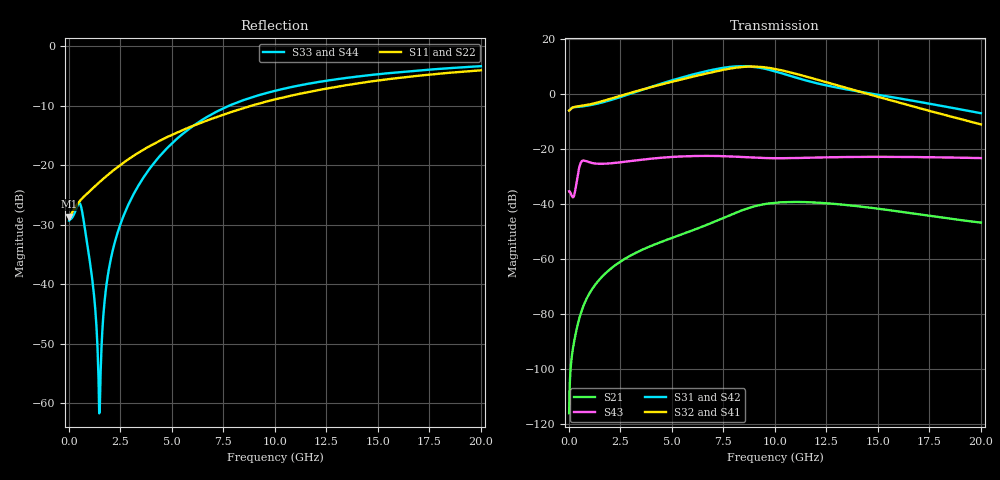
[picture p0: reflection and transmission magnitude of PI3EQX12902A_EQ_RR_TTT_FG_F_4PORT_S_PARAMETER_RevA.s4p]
! NPort=4 DATA=2000 NOISE=0 GROUPDELAY=0 COMPLEX_DATAFORMAT=POLAR
! NumOfBlock=1 NumOfParam=0
! .MODEL Smodel S TSTONEFILE=PI3EQX12902A_EQ_RR_TTT_FG_F_4PORT_S_PARAMETER_RevA.s4p TYPE=S
!  -- The above .MODEL line can be used for the S element in the netlist.
! The s parameter is extracted from the linear redriver, it is not bi-directional; only s(4,1)s(4,2) and s(3,1)s(3,2)
! should be the insertion loss
!Port definition:
!Port1 = input+
!Port2 = input-
!Port3 = output+
!Port4 = output-
# Hz S MA R  50
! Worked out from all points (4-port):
!   2000 points, 10 MHz to 20 GHz, reference 50 ohm
!   strongest paths, dB at 10 MHz, 5.01 GHz, 10.01 GHz, 15.01 GHz, 20 GHz:
!     S32: -6.0, 4.4, 9.1, -1.1, -11.1
!     S41: -6.0, 4.4, 9.0, -1.1, -11.0
!     S31: -6.0, 4.9, 8.2, -0.3, -7.0
!     S42: -6.0, 4.8, 8.0, -0.5, -7.1
!     S43: -35.3, -22.9, -23.4, -22.9, -23.3
!     S21: -116.0, -52.3, -39.5, -41.7, -46.7
!   lowest |S11| = -28.6 dB at 10 MHz (marker M1), VSWR 1.08, Z = 46.4 - j0.0607 ohm
!   |S11| at or under -10 dB: start of sweep to 8.865 GHz
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1e7  0.03704 -179.0  1.588e-06 51.9  0 0.0  0 0.0
     1.588e-06 51.9  0.03704 -179.0  0 0.0  0 0.0
     0.4994 0.9  0.4994 -179.1  0.03429 6.0  0.01709 -177.1
     0.4994 -179.1  0.4994 0.9  0.01709 -177.1  0.03429 6.0
1.49e9  0.07219 -133.4  0.0004295 116.7  3.743e-09 177.2  5.625e-09 -173.9
        0.0004295 116.7  0.07219 -133.4  5.627e-09 -173.8  3.745e-09 177.2
        0.6812 8.4  0.7154 -177.2  0.0008858 -60.3  0.05389 -174.9
        0.7133 -177.3  0.6809 8.1  0.05389 -174.8  0.0009453 -62.8
6.05e9  0.2147 -112.1  0.003385 89.6  1.739e-06 -24.9  1.079e-06 86.1
        0.003382 89.5  0.2147 -112.1  1.08e-06 86.2  1.73e-06 -24.6
        2.272 -46.4  2.069 109.2  0.215 -47.0  0.07411 144.1
        2.061 109.2  2.235 -47.0  0.07451 144.2  0.2143 -47.0
9.27e9  0.3314 -113.3  0.009643 47.3  1.159e-05 -124.8  8.967e-06 -7.7
        0.009602 47.4  0.3314 -113.3  8.935e-06 -7.7  1.156e-05 -124.0
        2.988 -144.7  3.1 6.2  0.3897 -76.2  0.06856 114.6
        3.067 6.3  2.919 -144.9  0.06899 114.4  0.3893 -76.1
1.096e10  0.3899 -115.8  0.01099 11.2  1.67e-05 -166.3  1.433e-05 -67.5
          0.01095 11.5  0.3899 -115.8  1.422e-05 -67.3  1.677e-05 -165.3
          2.01 170.9  2.349 -51.1  0.4601 -87.2  0.0682 105.6
          2.32 -50.7  1.956 170.9  0.06845 105.3  0.4602 -87.1
1.35e10  0.4717 -120.1  0.009595 -28.3  2.62e-05 148.1  1.857e-05 -137.4
         0.009587 -27.8  0.4718 -120.1  1.837e-05 -137.0  2.65e-05 148.7
         1.205 131.5  1.277 -114.5  0.5418 -99.7  0.07151 88.9
         1.266 -113.7  1.177 132.2  0.07149 88.6  0.5422 -99.6
2e10  0.6269 -131.5  0.00453 -72.3  4.311e-05 50.2  1.775e-05 103.3
      0.004612 -72.1  0.6269 -131.6  1.751e-05 104.7  4.373e-05 50.3
      0.4463 43.0  0.2797 135.3  0.6794 -119.6  0.06847 46.2
      0.2803 136.3  0.4421 43.8  0.06838 46.1  0.6797 -119.6
